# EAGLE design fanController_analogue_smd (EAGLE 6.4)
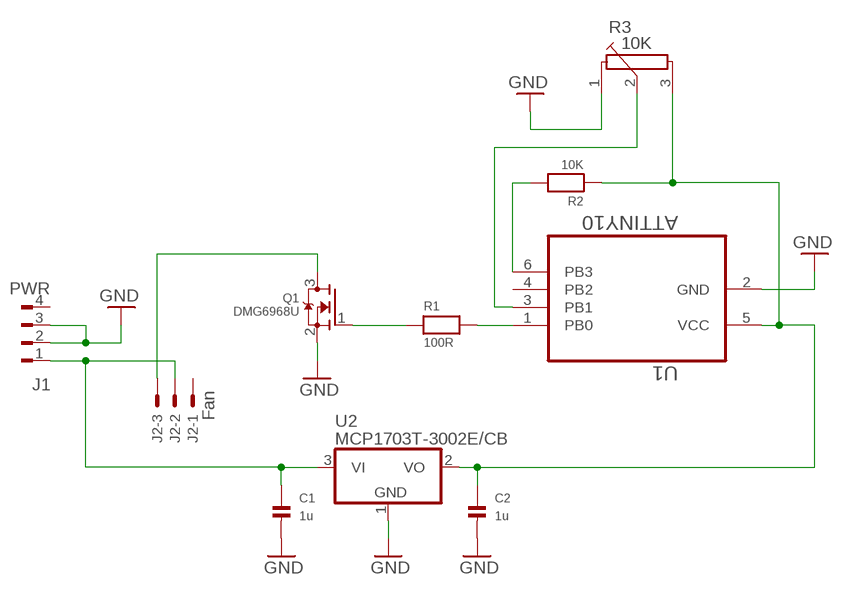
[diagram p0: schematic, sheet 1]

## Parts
C1  1u  CAP_CERAMIC0805-NOTHERMALS  [0805_NOTHERMALS]
C2  1u  CAP_CERAMIC0805-NOTHERMALS  [0805_NOTHERMALS]
J1  PWR  FLOP-4W827001  [827001]
J2  Fan  22-23-2031  [22-23-2031]
Q1  DMG6968U  MOSFET-NWAVE  [SOT23-W]
R1  100R  RESISTOR0805_NOTHERMALS  [0805_NOTHERMALS]
R2  10K  RESISTOR0805_NOTHERMALS  [0805_NOTHERMALS]
R3  10K  POTENTIOMETER  [POTENTIOMETER]
U1  ATTINY10  [SOT95P280X145-6N]
U2  MCP1703T-3002E/CB  MCP1703CB  [SOT23]

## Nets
GND: C1.2 C2.2 J1.2 J1.3 Q1.2(S) R3.1(1A) U1.2(GND) U2.1(GND)
HS: J2.3 Q1.3(D)
N$1: Q1.1(G) R1.1
N$2: C1.1 J1.1 J2.2 U2.3(VI)
N$3: R3.2(1S) U1.3(PB1)
N$6: R1.2 U1.1(PB0)
RST: R2.2 U1.6(PB3)
VCC: C2.1 R2.1 R3.3(1E) U1.5(VCC) U2.2(VO)
Unconnected: J1.4 J2.1 U1.4(PB2)

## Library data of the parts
C1 C2 = microbuilder:CAP_CERAMIC: Ceramic Capacitors
J1 = con-amp:FLOP-4W: MATE N-LOCK Floppy / HDD conector Distributor: Bürklin 71F972
J2 = con-molex:22-23-2031: .100" (2.54mm) Center Header - 3 Pin; MF: MOLEX; MPN: 22-23-2031; OC_FARNELL: 1462950; OC_NEWARK: 30C0862
Q1 = microbuilder:MOSFET-N: N-Channel Mosfet LEGEND VDS: Voltage Drain-Source ID: Drain Current RDS(ON): Drain-Source On-State Resistance VGS(TH): Gate-Source Threshold Voltage CISS: Drain-Source Input Capacitance SOT-23 Name VDS ID RDS(ON) VGS(TH) CISS Order Number 2N7002E 60V 260mA 2.5 Ohm 2.5V @ 250uA 26.7pF @ 25V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
R1 R2 = microbuilder:RESISTOR: Resistors
R3 = zak:POTENTIOMETER
U1 = zak:ATTINY10
U2 = linear:MCP1703: 250 mA, 16V, Low Quiescent Current LDO Regulator Source: http://ww1.microchip.com/downloads/en/DeviceDoc/22049b.pdf

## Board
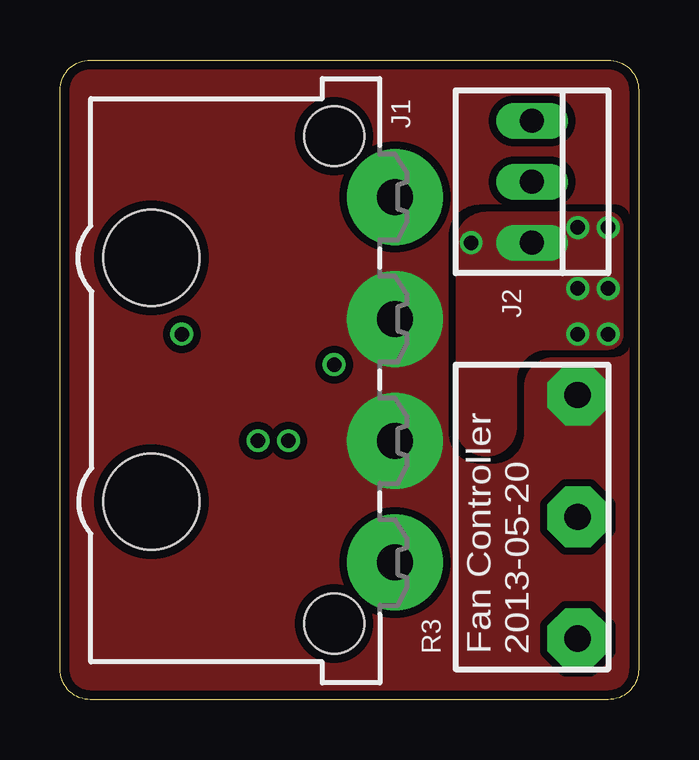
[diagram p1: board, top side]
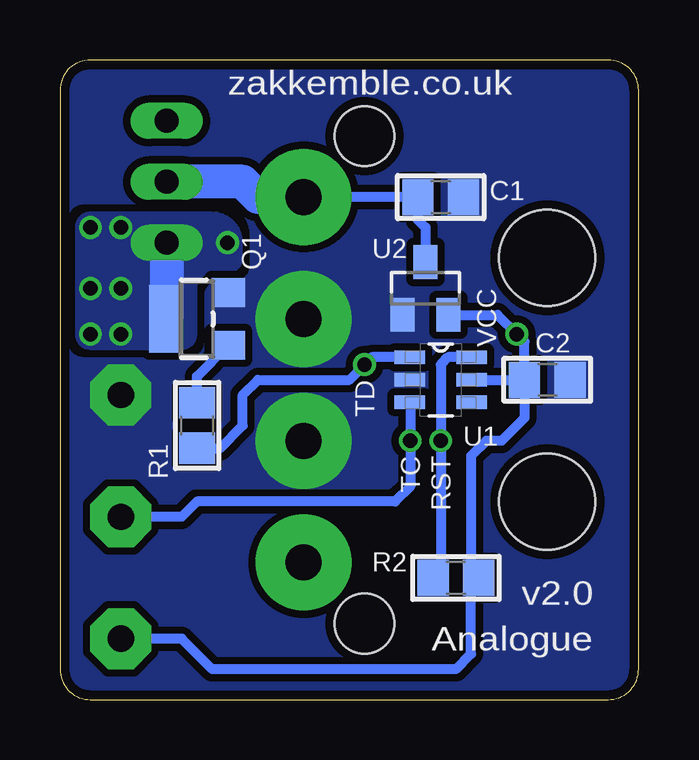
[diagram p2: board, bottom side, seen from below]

Size 24.13 x 26.67 mm. Coordinates in mm from the lower left corner, seen from the top.
Outline: 0,1.27 0,25.4 arc-90 1.27,26.67 22.86,26.67 arc-90 24.13,25.4 24.13,1.27 arc-90 22.86,0 1.27,0 arc-90 0,1.27
Copper layers (1*16): Top 0.0356mm / dielectric 1.5011mm / Bottom 0.0356mm
Design rules "default *": minimum track width 6mil, minimum drill 13mil, track to track 6mil, track to pad 6mil, pad to pad 6mil, via to via 6mil, smd to smd 6mil, copper to edge 15mil, drill to drill 6mil, minimum pad ring 10mil, minimum via ring 7mil, stop-mask expansion 4mil, vias tented up to drill 26mil, thermal gap 10mil

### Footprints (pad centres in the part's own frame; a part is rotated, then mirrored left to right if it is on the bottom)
0805_NOTHERMALS = smd 1.3 x 1.5: 1 -0.95,0; 2 0.95,0
827001 = drill 1.5 pad 4: 1 -7.62,0; 2 -2.54,0; 3 2.54,0; 4 7.62,0 | hole 4: 5.08,-10.16; -5.08,-10.16 | hole 2.5: 10.16,-2.54; -10.16,-2.54
22-23-2031 = drill 1 long: 1 -2.54,0; 2 0,0; 3 2.54,0
SOT23-W = smd 1.2 x 1.4: 1 -1.1,-1.3; 2 1.1,-1.3 | smd 2.8 x 1.4: 3 0,1.3
POTENTIOMETER = drill 1.1 pad 2.54 octagon: 1 1.905,5.08; 2 1.905,0; 3 1.905,-5.08
SOT95P280X145-6N = smd 1.27 x 0.559: 1 -1.295,0.94; 2 -1.295,0; 3 -1.295,-0.94; 4 1.295,-0.94; 5 1.295,0; 6 1.295,0.94
SOT23 = smd 1 x 1.4: 1 -0.95,-1.1; 2 0.95,-1.1; 3 0,1.1

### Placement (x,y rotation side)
C1  8.26,20.95 0 bottom
C2  3.81,13.34 0 bottom
J1  13.97,13.34 270 top
J2  19.68,21.59 270 top
Q1  18.41,15.88 90 bottom
R1  18.41,11.43 270 bottom
R2  7.62,5.08 180 bottom
R3  19.68,7.62 0 top
U1  8.26,13.34 0 bottom
U2  8.89,17.14 0 bottom

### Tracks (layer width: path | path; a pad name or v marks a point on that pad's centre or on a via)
GND
  pour Bottom (isolate 0.305, rank 6, no thermals): 0,26.67 24.13,26.67 24.13,0 0,0
  pour Top (isolate 0.305, rank 6, no thermals): 0,26.67 24.13,26.67 24.13,0 0,0
HS  (via drill 0.6)
  Bottom 1.422: J2.3 19.68,15.9 Q1.3
  other vias: 22.86,17.14 22.86,15.24 21.59,15.24 21.59,17.14 22.86,19.68 21.59,19.68 17.14,19.05
  pour Top (isolate 0.305, no thermals): 22.86,20.32 17.78,20.32 arc90 16.51,19.05 16.51,11.43 arc90 17.78,10.16 arc90 19.05,11.43 19.05,13.34 arc-90 20.32,14.61 22.86,14.61 arc90 23.5,15.24 23.5,19.68 arc90
  pour Bottom (isolate 0.305, no thermals): 23.5,15.24 arc-90 22.86,14.61 19.05,14.61 arc-90 18.41,15.24 18.41,17.14 arc90 17.78,17.78 17.14,17.78 arc-90 16.51,18.41 16.51,19.05 arc-90 17.78,20.32 22.86,20.32 arc-90 23.5,19.68
N$1
  Bottom 0.406: R1.1 18.41,13.47 Q1.1
N$2
  Bottom 0.406: J1.1 C1.1 9.21,20 8.89,19.68 U2.3
  Bottom 1.422: J1.1 15.88,20.95 16.51,21.59 J2.2
N$3  (via drill 0.6)
  Bottom 0.406: U1.3 9.53,12.37 v9.53,10.79 9.53,8.89 10.16,8.26 18.41,8.26 19.05,7.62 R3.2
N$6  (via drill 0.6)
  Bottom 0.406: R1.2 17.46,10.48 16.51,11.43 16.51,12.7 15.88,13.34 12.06,13.34 v11.43,13.97 11.12,14.28 U1.1
RST  (via drill 0.6)
  Bottom 0.406: U1.6 7.95,14.28 8.26,13.97 v8.26,10.79 8.26,5.39 R2.2
VCC  (via drill 0.6)
  Bottom 0.406: U1.5 C2.1 | U2.2 5.88,16.05 v5.08,15.24 4.76,14.92 C2.1 | C2.1 4.76,11.75 5.71,10.79 6.35,10.79 6.99,10.16 6.99,5.39 R2.1 6.99,4.76 6.99,1.91 7.62,1.27 17.78,1.27 19.05,2.54 R3.3

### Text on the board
tPlace: Fan Controller | 2013-05-20
bPlace: zakkemble.co.uk | VCC | TD | RST | TC | v2.0 | Analogue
